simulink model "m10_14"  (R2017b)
settings: Solver=VariableStepAuto  StartTime=0.0  StopTime=10.0  RelTol=1e-3

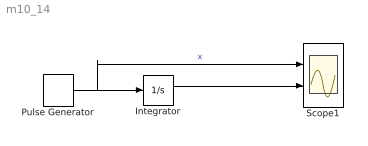
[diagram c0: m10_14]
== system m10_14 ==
  Integrator : Integrator
  Pulse Generator : DiscretePulseGenerator  PulseType=Time based  PulseWidth=50
  Scope1 : Scope  NumInputPorts=2
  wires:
  Pulse Generator/1 -> Scope1/1, Integrator/1  "x"
  Integrator/1 -> Scope1/2
